(* Logix 5000 AddOnInstructionDefinition export Banner_QS18EAF_Param_v4; software revision 33.00; part 2 of 2 *)
(* tags used below, declared in another part *)
   QS18EAF : Banner_QS18EAF_v4;
   Port_Data : Banner_IOL_Port_v4;
   Port : DINT;
   Local_Control : DINT;
   Command_Being_Processed : BOOL;
   Update_Archive : BOOL;
   Index_Write_Inprocess : INT;
   Index_Write_Control : INT;
   Inprocess_Index : DINT;
(* Banner_QS18EAF_Param_v4, continued *)

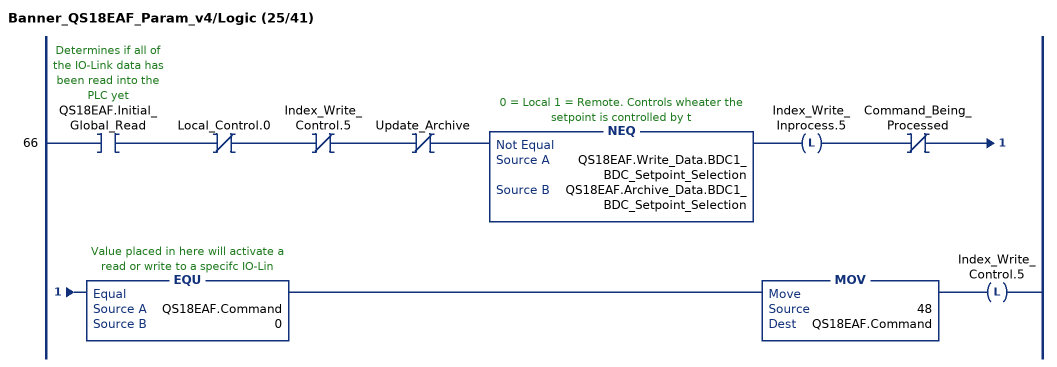
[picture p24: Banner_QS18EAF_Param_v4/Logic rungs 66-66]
   66: XIC(QS18EAF.Initial_Global_Read)XIO(Local_Control.0)XIO(Index_Write_Control.5)XIO(Update_Archive)NEQ(QS18EAF.Write_Data.BDC1_BDC_Setpoint_Selection,QS18EAF.Archive_Data.BDC1_BDC_Setpoint_Selection)OTL(Index_Write_Inprocess.5)XIO(Command_Being_Processed)EQU(QS18EAF.Command,0)MOV(48,QS18EAF.Command)OTL(Index_Write_Control.5);
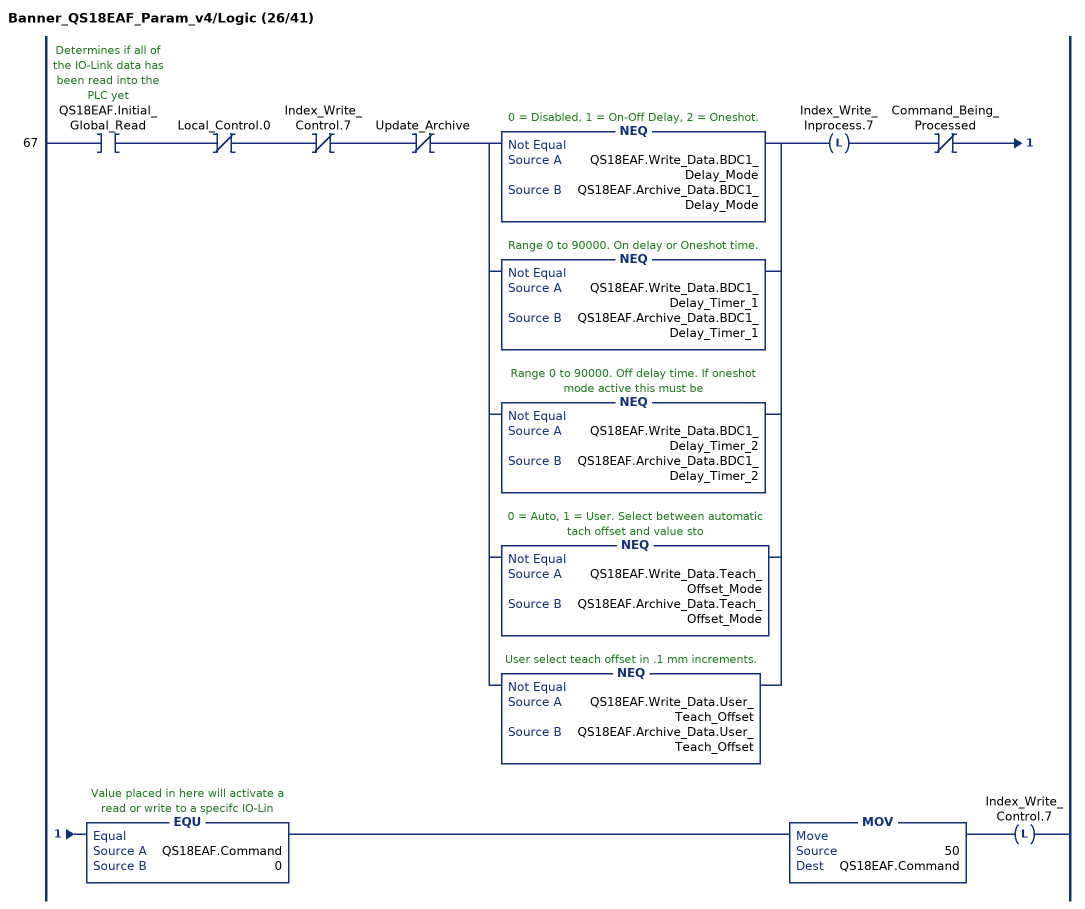
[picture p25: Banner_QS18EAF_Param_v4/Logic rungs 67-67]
   67: XIC(QS18EAF.Initial_Global_Read)XIO(Local_Control.0)XIO(Index_Write_Control.7)XIO(Update_Archive)[NEQ(QS18EAF.Write_Data.BDC1_Delay_Mode,QS18EAF.Archive_Data.BDC1_Delay_Mode) ,NEQ(QS18EAF.Write_Data.BDC1_Delay_Timer_1,QS18EAF.Archive_Data.BDC1_Delay_Timer_1) ,NEQ(QS18EAF.Write_Data.BDC1_Delay_Timer_2,QS18EAF.Archive_Data.BDC1_Delay_Timer_2) ,NEQ(QS18EAF.Write_Data.Teach_Offset_Mode,QS18EAF.Archive_Data.Teach_Offset_Mode) ,NEQ(QS18EAF.Write_Data.User_Teach_Offset,QS18EAF.Archive_Data.User_Teach_Offset) ]OTL(Index_Write_Inprocess.7)XIO(Command_Being_Processed)EQU(QS18EAF.Command,0)MOV(50,QS18EAF.Command)OTL(Index_Write_Control.7);
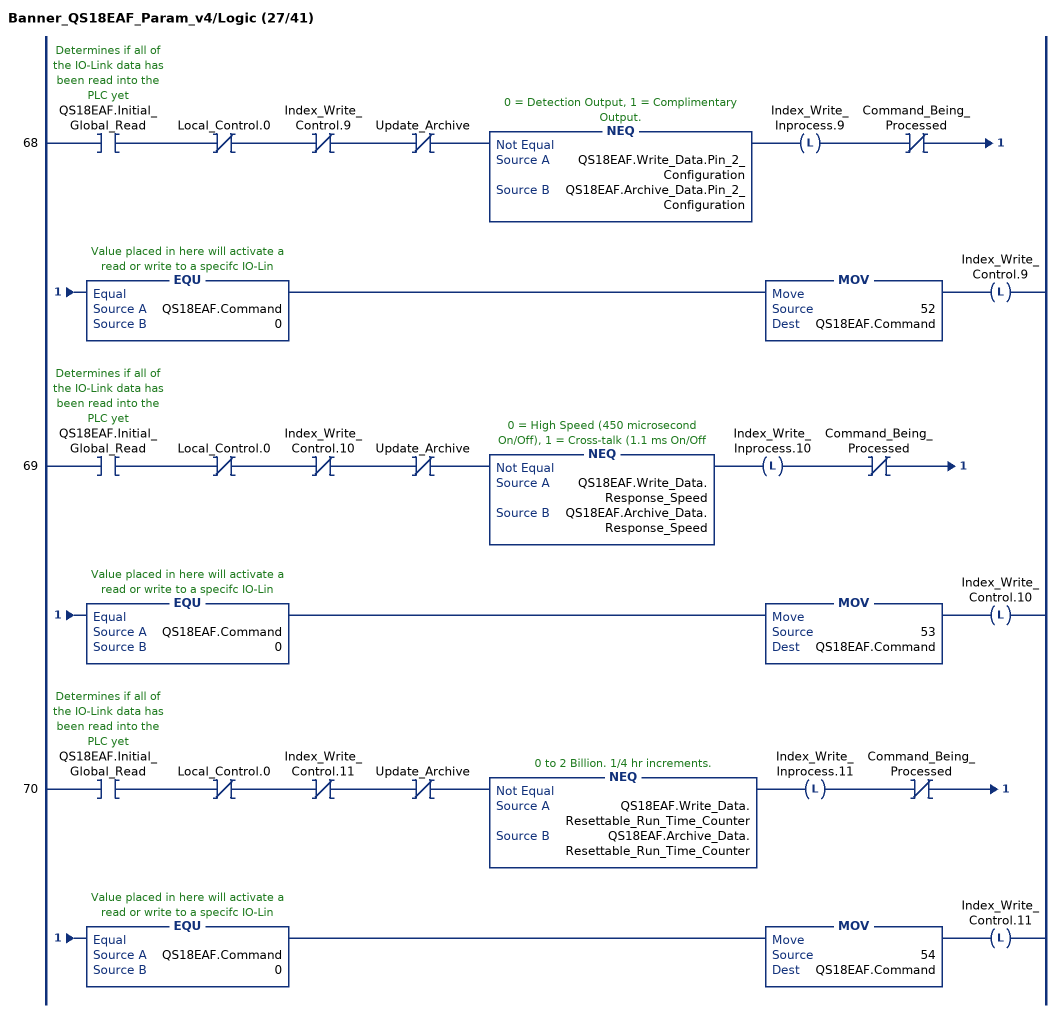
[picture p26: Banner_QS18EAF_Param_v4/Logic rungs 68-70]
   68: XIC(QS18EAF.Initial_Global_Read)XIO(Local_Control.0)XIO(Index_Write_Control.9)XIO(Update_Archive)NEQ(QS18EAF.Write_Data.Pin_2_Configuration,QS18EAF.Archive_Data.Pin_2_Configuration)OTL(Index_Write_Inprocess.9)XIO(Command_Being_Processed)EQU(QS18EAF.Command,0)MOV(52,QS18EAF.Command)OTL(Index_Write_Control.9);
   69: XIC(QS18EAF.Initial_Global_Read)XIO(Local_Control.0)XIO(Index_Write_Control.10)XIO(Update_Archive)NEQ(QS18EAF.Write_Data.Response_Speed,QS18EAF.Archive_Data.Response_Speed)OTL(Index_Write_Inprocess.10)XIO(Command_Being_Processed)EQU(QS18EAF.Command,0)MOV(53,QS18EAF.Command)OTL(Index_Write_Control.10);
   70: XIC(QS18EAF.Initial_Global_Read)XIO(Local_Control.0)XIO(Index_Write_Control.11)XIO(Update_Archive)NEQ(QS18EAF.Write_Data.Resettable_Run_Time_Counter,QS18EAF.Archive_Data.Resettable_Run_Time_Counter)OTL(Index_Write_Inprocess.11)XIO(Command_Being_Processed)EQU(QS18EAF.Command,0)MOV(54,QS18EAF.Command)OTL(Index_Write_Control.11);
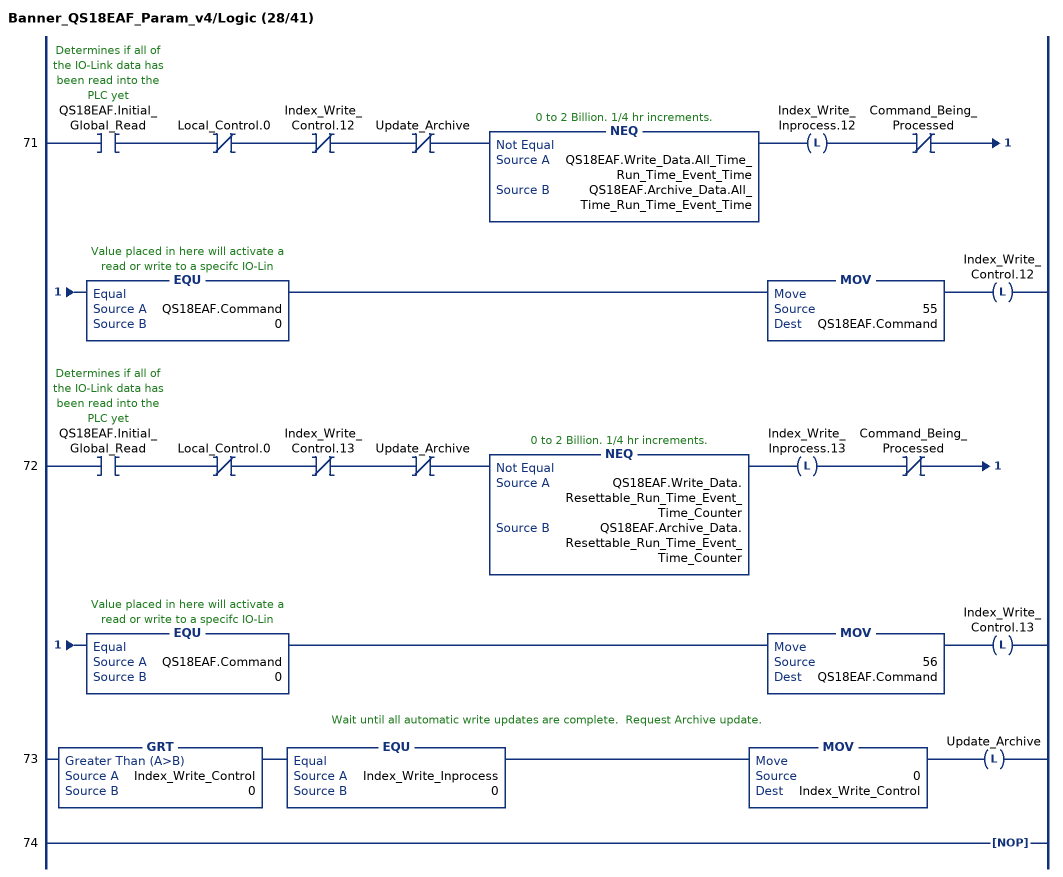
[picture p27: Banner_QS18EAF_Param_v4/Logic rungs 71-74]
   71: XIC(QS18EAF.Initial_Global_Read)XIO(Local_Control.0)XIO(Index_Write_Control.12)XIO(Update_Archive)NEQ(QS18EAF.Write_Data.All_Time_Run_Time_Event_Time,QS18EAF.Archive_Data.All_Time_Run_Time_Event_Time)OTL(Index_Write_Inprocess.12)XIO(Command_Being_Processed)EQU(QS18EAF.Command,0)MOV(55,QS18EAF.Command)OTL(Index_Write_Control.12);
   72: XIC(QS18EAF.Initial_Global_Read)XIO(Local_Control.0)XIO(Index_Write_Control.13)XIO(Update_Archive)NEQ(QS18EAF.Write_Data.Resettable_Run_Time_Event_Time_Counter,QS18EAF.Archive_Data.Resettable_Run_Time_Event_Time_Counter)OTL(Index_Write_Inprocess.13)XIO(Command_Being_Processed)EQU(QS18EAF.Command,0)MOV(56,QS18EAF.Command)OTL(Index_Write_Control.13);
   // Wait until all automatic write updates are complete.  Request Archive update.
   73: GRT(Index_Write_Control,0)EQU(Index_Write_Inprocess,0)MOV(0,Index_Write_Control)OTL(Update_Archive);
   74: NOP();
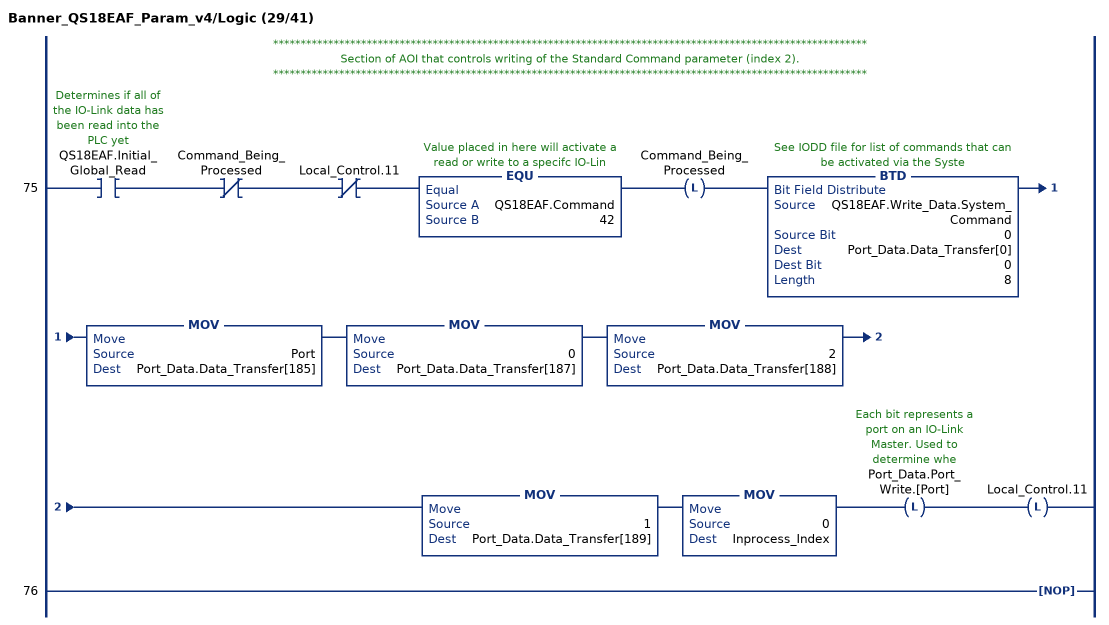
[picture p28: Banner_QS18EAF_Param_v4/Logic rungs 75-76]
   // ************************************************************************************************************
   // Section of AOI that controls writing of the Standard Command parameter (index 2).
   // ************************************************************************************************************
   75: XIC(QS18EAF.Initial_Global_Read)XIO(Command_Being_Processed)XIO(Local_Control.11)EQU(QS18EAF.Command,42)OTL(Command_Being_Processed)BTD(QS18EAF.Write_Data.System_Command,0,Port_Data.Data_Transfer[0],0,8)MOV(Port,Port_Data.Data_Transfer[185])MOV(0,Port_Data.Data_Transfer[187])MOV(2,Port_Data.Data_Transfer[188])MOV(1,Port_Data.Data_Transfer[189])MOV(0,Inprocess_Index)OTL(Port_Data.Port_Write.[Port])OTL(Local_Control.11);
   76: NOP();
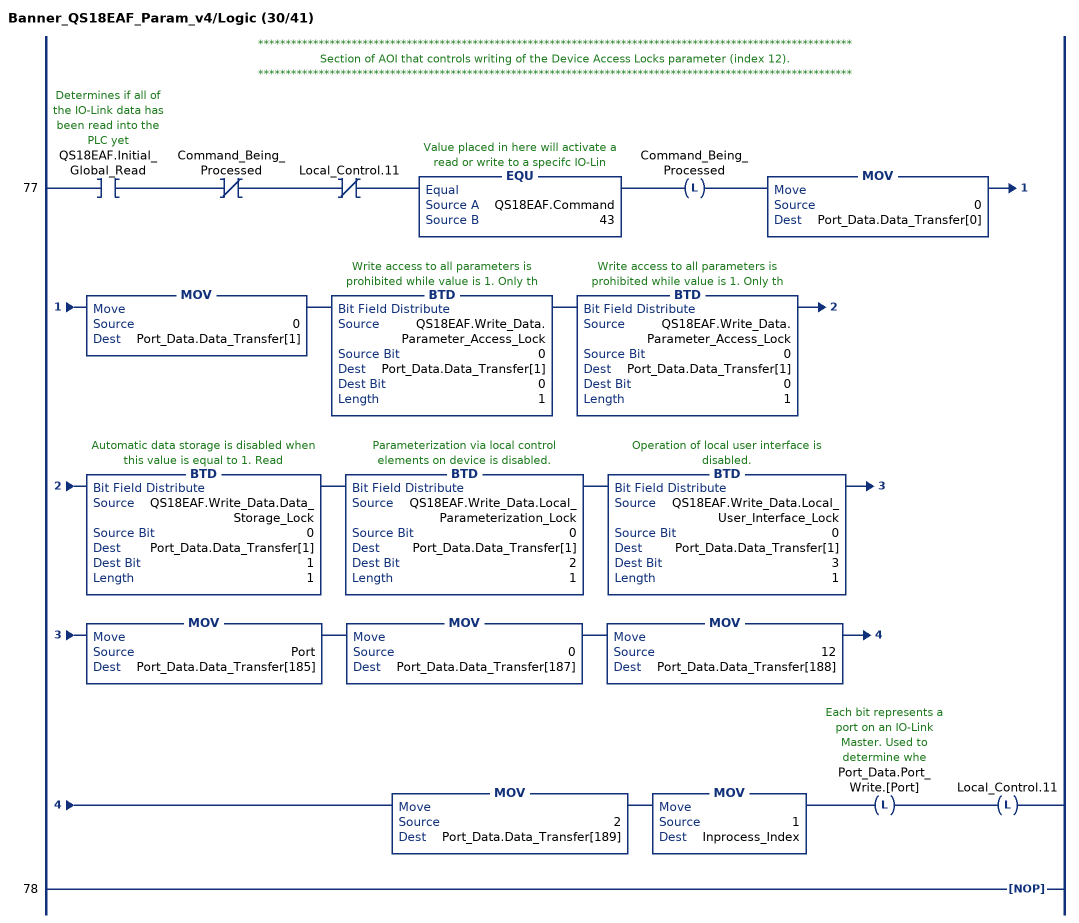
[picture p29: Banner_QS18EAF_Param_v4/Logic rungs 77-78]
   // ************************************************************************************************************
   // Section of AOI that controls writing of the Device Access Locks parameter (index 12).
   // ************************************************************************************************************
   77: XIC(QS18EAF.Initial_Global_Read)XIO(Command_Being_Processed)XIO(Local_Control.11)EQU(QS18EAF.Command,43)OTL(Command_Being_Processed)MOV(0,Port_Data.Data_Transfer[0])MOV(0,Port_Data.Data_Transfer[1])BTD(QS18EAF.Write_Data.Parameter_Access_Lock,0,Port_Data.Data_Transfer[1],0,1)BTD(QS18EAF.Write_Data.Parameter_Access_Lock,0,Port_Data.Data_Transfer[1],0,1)BTD(QS18EAF.Write_Data.Data_Storage_Lock,0,Port_Data.Data_Transfer[1],1,1)BTD(QS18EAF.Write_Data.Local_Parameterization_Lock,0,Port_Data.Data_Transfer[1],2,1)BTD(QS18EAF.Write_Data.Local_User_Interface_Lock,0,Port_Data.Data_Transfer[1],3,1)MOV(Port,Port_Data.Data_Transfer[185])MOV(0,Port_Data.Data_Transfer[187])MOV(12,Port_Data.Data_Transfer[188])MOV(2,Port_Data.Data_Transfer[189])MOV(1,Inprocess_Index)OTL(Port_Data.Port_Write.[Port])OTL(Local_Control.11);
   78: NOP();
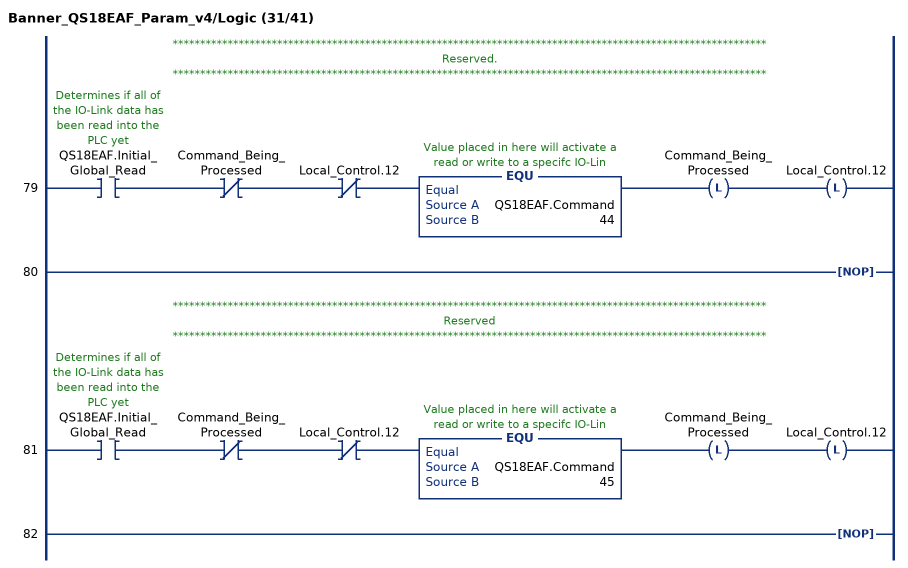
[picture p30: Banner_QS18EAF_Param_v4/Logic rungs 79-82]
   // ************************************************************************************************************
   // Reserved.
   // ************************************************************************************************************
   79: XIC(QS18EAF.Initial_Global_Read)XIO(Command_Being_Processed)XIO(Local_Control.12)EQU(QS18EAF.Command,44)OTL(Command_Being_Processed)OTL(Local_Control.12);
   80: NOP();
   // ************************************************************************************************************
   // Reserved
   // ************************************************************************************************************
   81: XIC(QS18EAF.Initial_Global_Read)XIO(Command_Being_Processed)XIO(Local_Control.12)EQU(QS18EAF.Command,45)OTL(Command_Being_Processed)OTL(Local_Control.12);
   82: NOP();
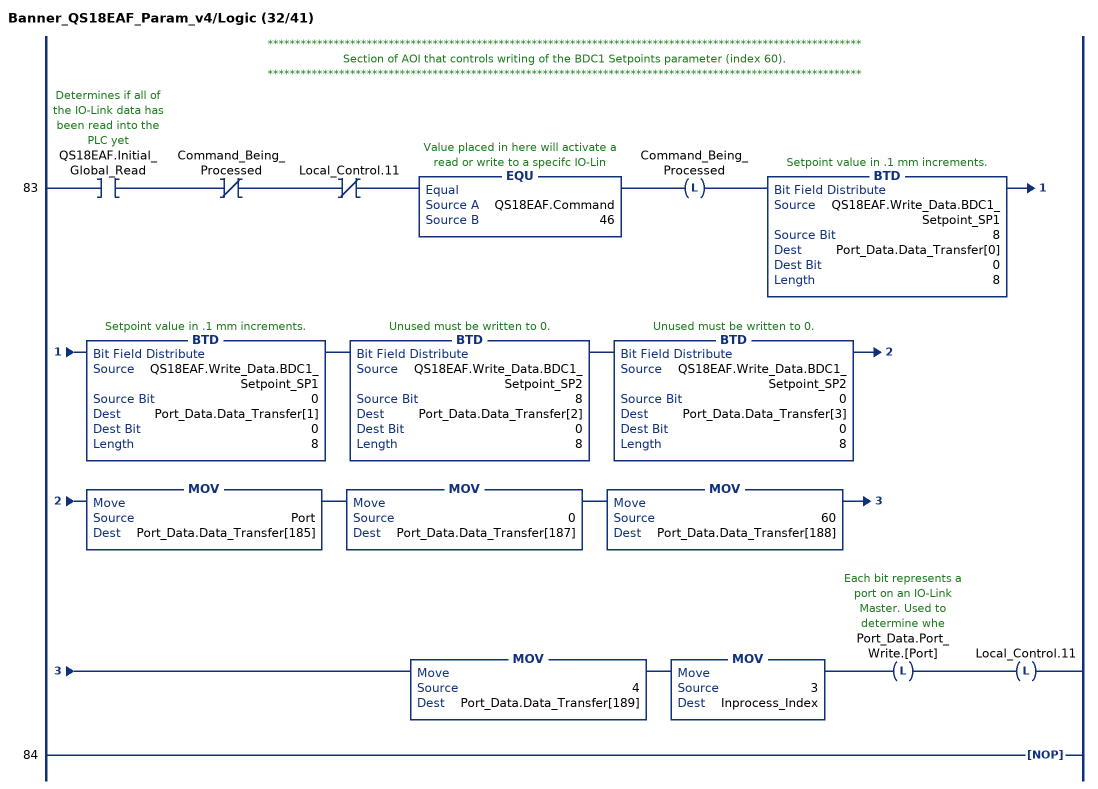
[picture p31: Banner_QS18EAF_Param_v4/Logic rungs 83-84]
   // ************************************************************************************************************
   // Section of AOI that controls writing of the BDC1 Setpoints parameter (index 60).
   // ************************************************************************************************************
   83: XIC(QS18EAF.Initial_Global_Read)XIO(Command_Being_Processed)XIO(Local_Control.11)EQU(QS18EAF.Command,46)OTL(Command_Being_Processed)BTD(QS18EAF.Write_Data.BDC1_Setpoint_SP1,8,Port_Data.Data_Transfer[0],0,8)BTD(QS18EAF.Write_Data.BDC1_Setpoint_SP1,0,Port_Data.Data_Transfer[1],0,8)BTD(QS18EAF.Write_Data.BDC1_Setpoint_SP2,8,Port_Data.Data_Transfer[2],0,8)BTD(QS18EAF.Write_Data.BDC1_Setpoint_SP2,0,Port_Data.Data_Transfer[3],0,8)MOV(Port,Port_Data.Data_Transfer[185])MOV(0,Port_Data.Data_Transfer[187])MOV(60,Port_Data.Data_Transfer[188])MOV(4,Port_Data.Data_Transfer[189])MOV(3,Inprocess_Index)OTL(Port_Data.Port_Write.[Port])OTL(Local_Control.11);
   84: NOP();
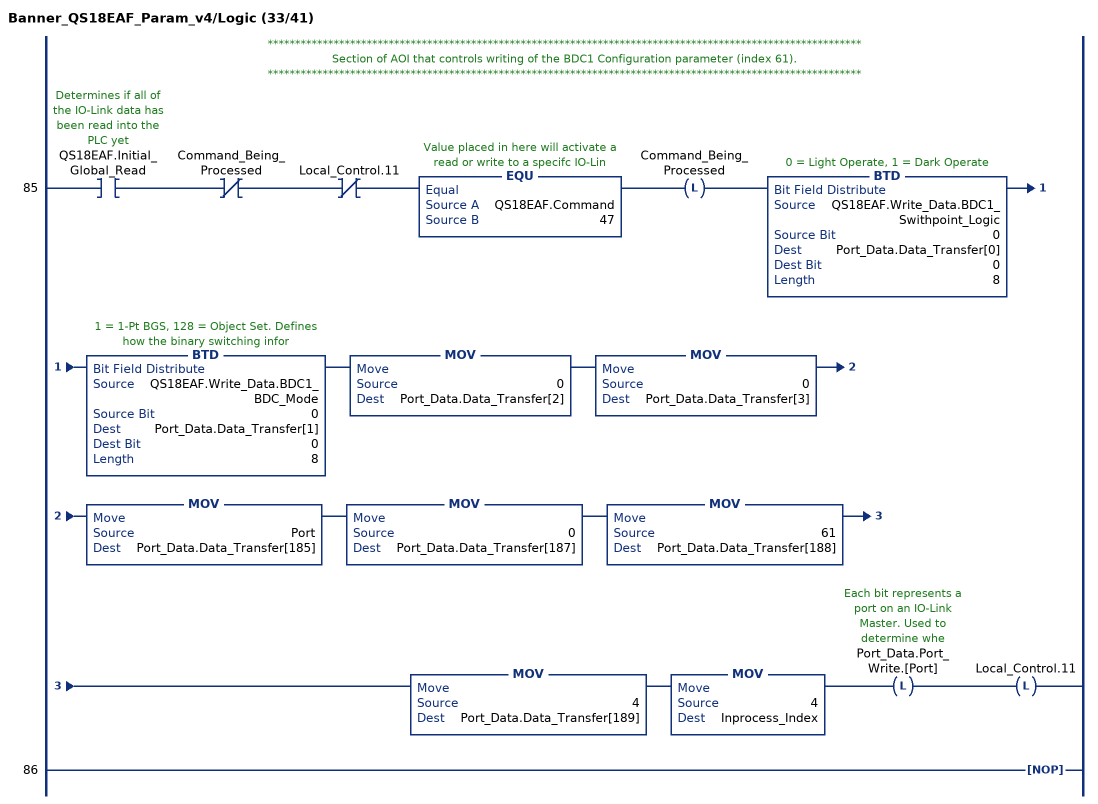
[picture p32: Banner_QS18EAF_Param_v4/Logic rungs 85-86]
   // ************************************************************************************************************
   // Section of AOI that controls writing of the BDC1 Configuration parameter (index 61).
   // ************************************************************************************************************
   85: XIC(QS18EAF.Initial_Global_Read)XIO(Command_Being_Processed)XIO(Local_Control.11)EQU(QS18EAF.Command,47)OTL(Command_Being_Processed)BTD(QS18EAF.Write_Data.BDC1_Swithpoint_Logic,0,Port_Data.Data_Transfer[0],0,8)BTD(QS18EAF.Write_Data.BDC1_BDC_Mode,0,Port_Data.Data_Transfer[1],0,8)MOV(0,Port_Data.Data_Transfer[2])MOV(0,Port_Data.Data_Transfer[3])MOV(Port,Port_Data.Data_Transfer[185])MOV(0,Port_Data.Data_Transfer[187])MOV(61,Port_Data.Data_Transfer[188])MOV(4,Port_Data.Data_Transfer[189])MOV(4,Inprocess_Index)OTL(Port_Data.Port_Write.[Port])OTL(Local_Control.11);
   86: NOP();
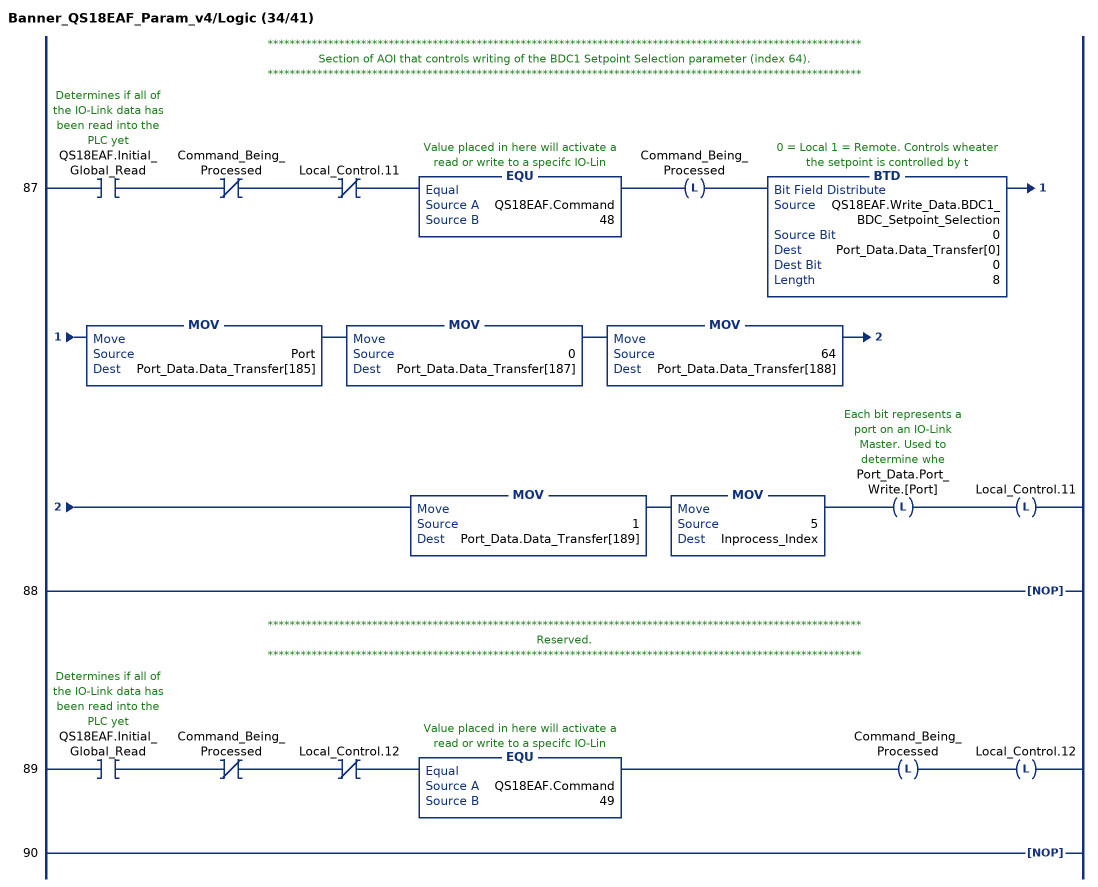
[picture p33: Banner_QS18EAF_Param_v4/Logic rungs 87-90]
   // ************************************************************************************************************
   // Section of AOI that controls writing of the BDC1 Setpoint Selection parameter (index 64).
   // ************************************************************************************************************
   87: XIC(QS18EAF.Initial_Global_Read)XIO(Command_Being_Processed)XIO(Local_Control.11)EQU(QS18EAF.Command,48)OTL(Command_Being_Processed)BTD(QS18EAF.Write_Data.BDC1_BDC_Setpoint_Selection,0,Port_Data.Data_Transfer[0],0,8)MOV(Port,Port_Data.Data_Transfer[185])MOV(0,Port_Data.Data_Transfer[187])MOV(64,Port_Data.Data_Transfer[188])MOV(1,Port_Data.Data_Transfer[189])MOV(5,Inprocess_Index)OTL(Port_Data.Port_Write.[Port])OTL(Local_Control.11);
   88: NOP();
   // ************************************************************************************************************
   // Reserved.
   // ************************************************************************************************************
   89: XIC(QS18EAF.Initial_Global_Read)XIO(Command_Being_Processed)XIO(Local_Control.12)EQU(QS18EAF.Command,49)OTL(Command_Being_Processed)OTL(Local_Control.12);
   90: NOP();
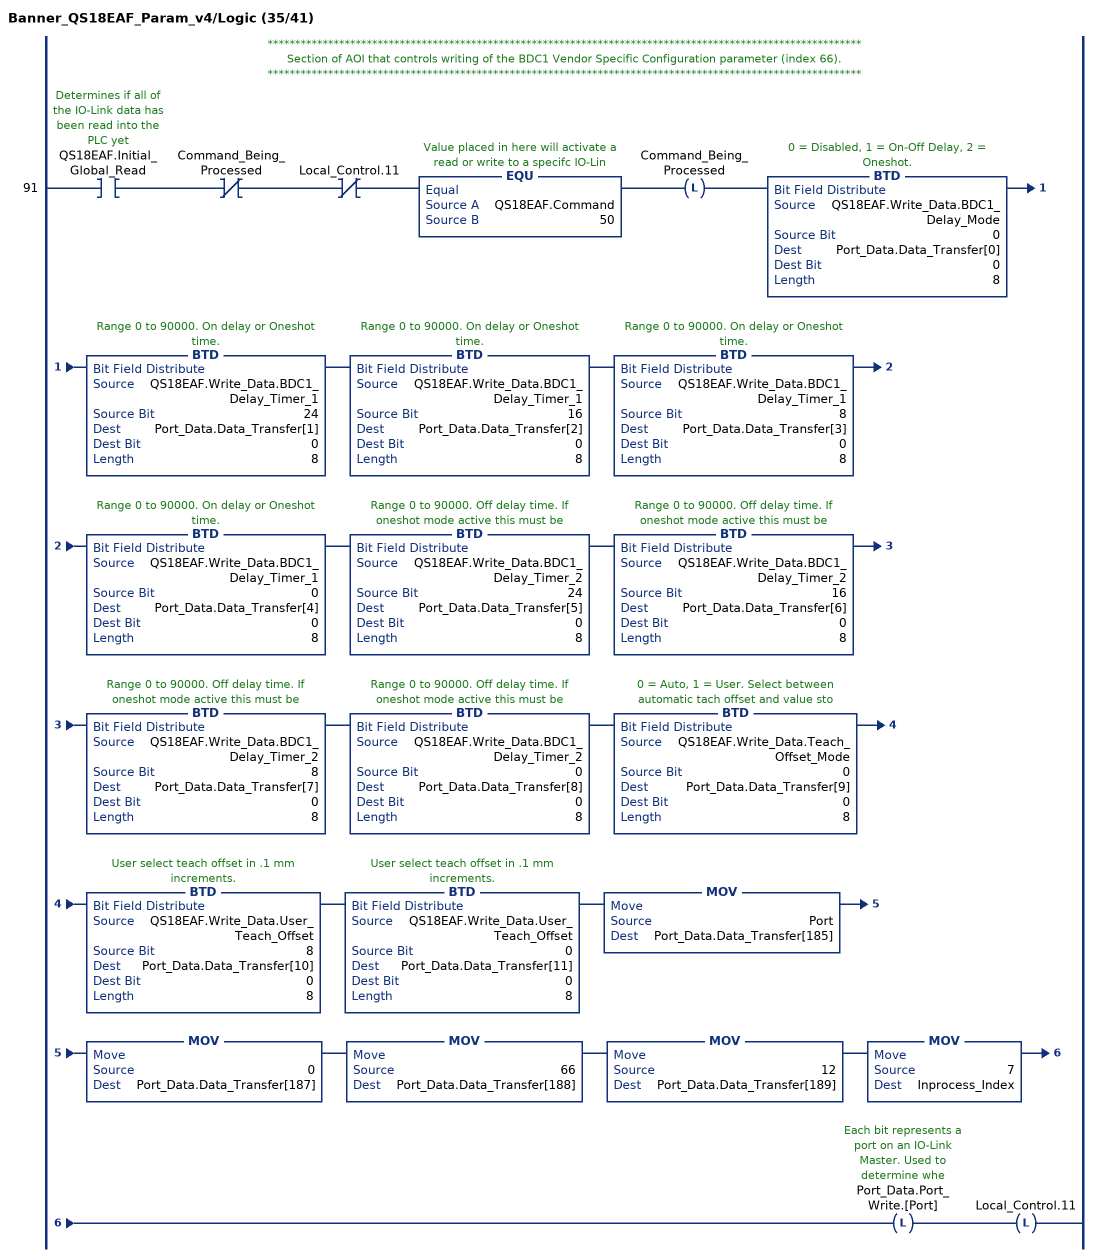
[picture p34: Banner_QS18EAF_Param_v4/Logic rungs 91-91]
   // ************************************************************************************************************
   // Section of AOI that controls writing of the BDC1 Vendor Specific Configuration parameter (index 66).
   // ************************************************************************************************************
   91: XIC(QS18EAF.Initial_Global_Read)XIO(Command_Being_Processed)XIO(Local_Control.11)EQU(QS18EAF.Command,50)OTL(Command_Being_Processed)BTD(QS18EAF.Write_Data.BDC1_Delay_Mode,0,Port_Data.Data_Transfer[0],0,8)BTD(QS18EAF.Write_Data.BDC1_Delay_Timer_1,24,Port_Data.Data_Transfer[1],0,8)BTD(QS18EAF.Write_Data.BDC1_Delay_Timer_1,16,Port_Data.Data_Transfer[2],0,8)BTD(QS18EAF.Write_Data.BDC1_Delay_Timer_1,8,Port_Data.Data_Transfer[3],0,8)BTD(QS18EAF.Write_Data.BDC1_Delay_Timer_1,0,Port_Data.Data_Transfer[4],0,8)BTD(QS18EAF.Write_Data.BDC1_Delay_Timer_2,24,Port_Data.Data_Transfer[5],0,8)BTD(QS18EAF.Write_Data.BDC1_Delay_Timer_2,16,Port_Data.Data_Transfer[6],0,8)BTD(QS18EAF.Write_Data.BDC1_Delay_Timer_2,8,Port_Data.Data_Transfer[7],0,8)BTD(QS18EAF.Write_Data.BDC1_Delay_Timer_2,0,Port_Data.Data_Transfer[8],0,8)BTD(QS18EAF.Write_Data.Teach_Offset_Mode,0,Port_Data.Data_Transfer[9],0,8)BTD(QS18EAF.Write_Data.User_Teach_Offset,8,Port_Data.Data_Transfer[10],0,8)BTD(QS18EAF.Write_Data.User_Teach_Offset,0,Port_Data.Data_Transfer[11],0,8)MOV(Port,Port_Data.Data_Transfer[185])MOV(0,Port_Data.Data_Transfer[187])MOV(66,Port_Data.Data_Transfer[188])MOV(12,Port_Data.Data_Transfer[189])MOV(7,Inprocess_Index)OTL(Port_Data.Port_Write.[Port])OTL(Local_Control.11);
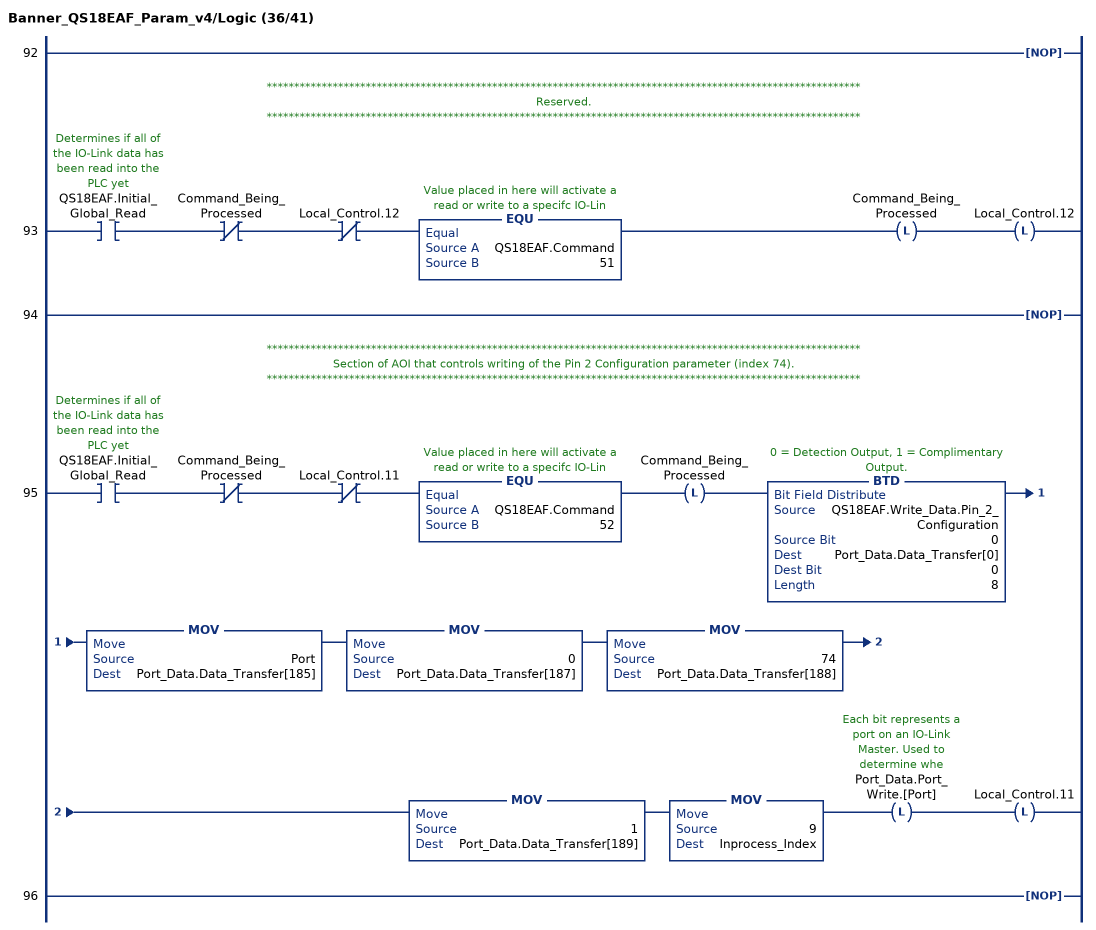
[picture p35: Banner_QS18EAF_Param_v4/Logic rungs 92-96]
   92: NOP();
   // ************************************************************************************************************
   // Reserved.
   // ************************************************************************************************************
   93: XIC(QS18EAF.Initial_Global_Read)XIO(Command_Being_Processed)XIO(Local_Control.12)EQU(QS18EAF.Command,51)OTL(Command_Being_Processed)OTL(Local_Control.12);
   94: NOP();
   // ************************************************************************************************************
   // Section of AOI that controls writing of the Pin 2 Configuration parameter (index 74).
   // ************************************************************************************************************
   95: XIC(QS18EAF.Initial_Global_Read)XIO(Command_Being_Processed)XIO(Local_Control.11)EQU(QS18EAF.Command,52)OTL(Command_Being_Processed)BTD(QS18EAF.Write_Data.Pin_2_Configuration,0,Port_Data.Data_Transfer[0],0,8)MOV(Port,Port_Data.Data_Transfer[185])MOV(0,Port_Data.Data_Transfer[187])MOV(74,Port_Data.Data_Transfer[188])MOV(1,Port_Data.Data_Transfer[189])MOV(9,Inprocess_Index)OTL(Port_Data.Port_Write.[Port])OTL(Local_Control.11);
   96: NOP();
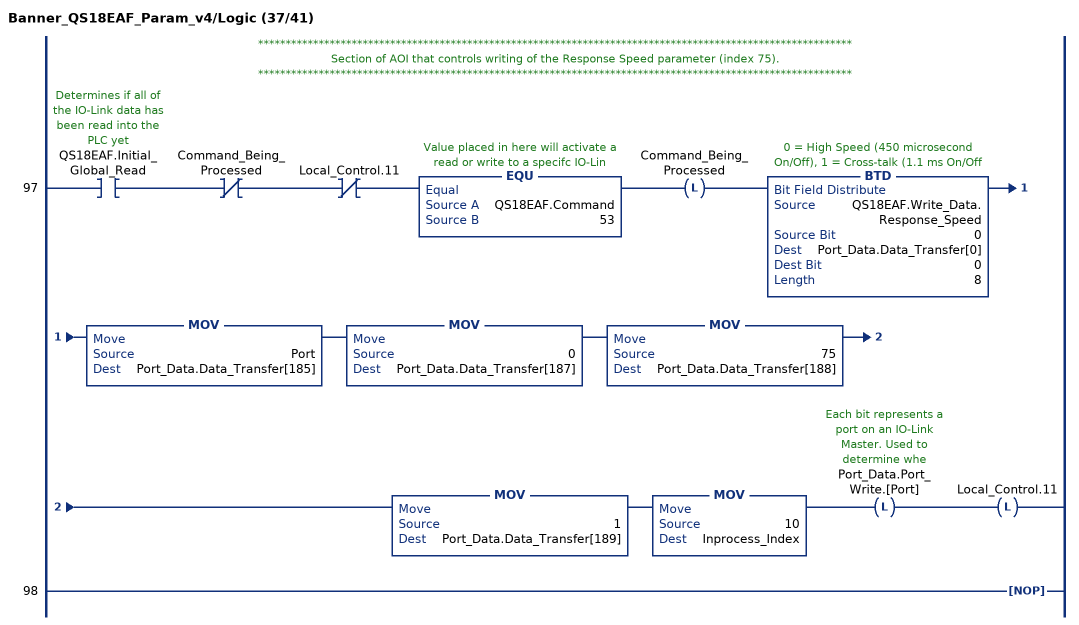
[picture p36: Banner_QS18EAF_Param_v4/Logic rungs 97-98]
   // ************************************************************************************************************
   // Section of AOI that controls writing of the Response Speed parameter (index 75).
   // ************************************************************************************************************
   97: XIC(QS18EAF.Initial_Global_Read)XIO(Command_Being_Processed)XIO(Local_Control.11)EQU(QS18EAF.Command,53)OTL(Command_Being_Processed)BTD(QS18EAF.Write_Data.Response_Speed,0,Port_Data.Data_Transfer[0],0,8)MOV(Port,Port_Data.Data_Transfer[185])MOV(0,Port_Data.Data_Transfer[187])MOV(75,Port_Data.Data_Transfer[188])MOV(1,Port_Data.Data_Transfer[189])MOV(10,Inprocess_Index)OTL(Port_Data.Port_Write.[Port])OTL(Local_Control.11);
   98: NOP();
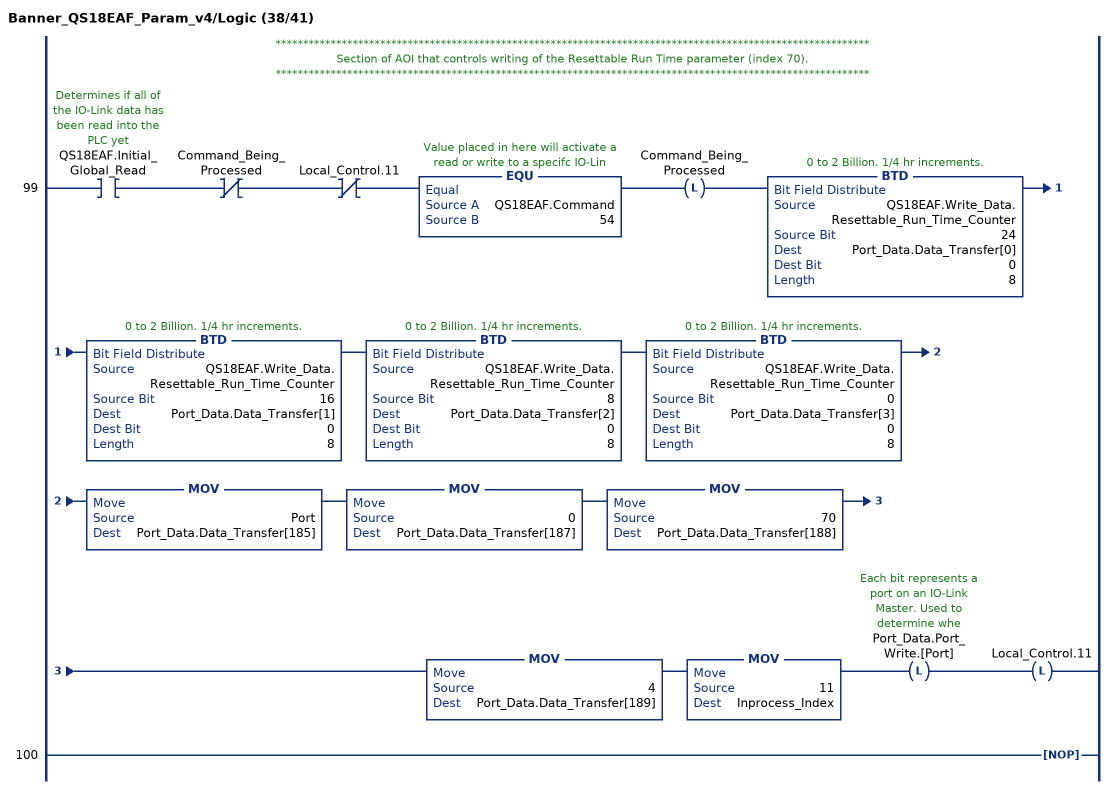
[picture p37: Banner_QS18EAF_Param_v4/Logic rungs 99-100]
   // ************************************************************************************************************
   // Section of AOI that controls writing of the Resettable Run Time parameter (index 70).
   // ************************************************************************************************************
   99: XIC(QS18EAF.Initial_Global_Read)XIO(Command_Being_Processed)XIO(Local_Control.11)EQU(QS18EAF.Command,54)OTL(Command_Being_Processed)BTD(QS18EAF.Write_Data.Resettable_Run_Time_Counter,24,Port_Data.Data_Transfer[0],0,8)BTD(QS18EAF.Write_Data.Resettable_Run_Time_Counter,16,Port_Data.Data_Transfer[1],0,8)BTD(QS18EAF.Write_Data.Resettable_Run_Time_Counter,8,Port_Data.Data_Transfer[2],0,8)BTD(QS18EAF.Write_Data.Resettable_Run_Time_Counter,0,Port_Data.Data_Transfer[3],0,8)MOV(Port,Port_Data.Data_Transfer[185])MOV(0,Port_Data.Data_Transfer[187])MOV(70,Port_Data.Data_Transfer[188])MOV(4,Port_Data.Data_Transfer[189])MOV(11,Inprocess_Index)OTL(Port_Data.Port_Write.[Port])OTL(Local_Control.11);
   100: NOP();
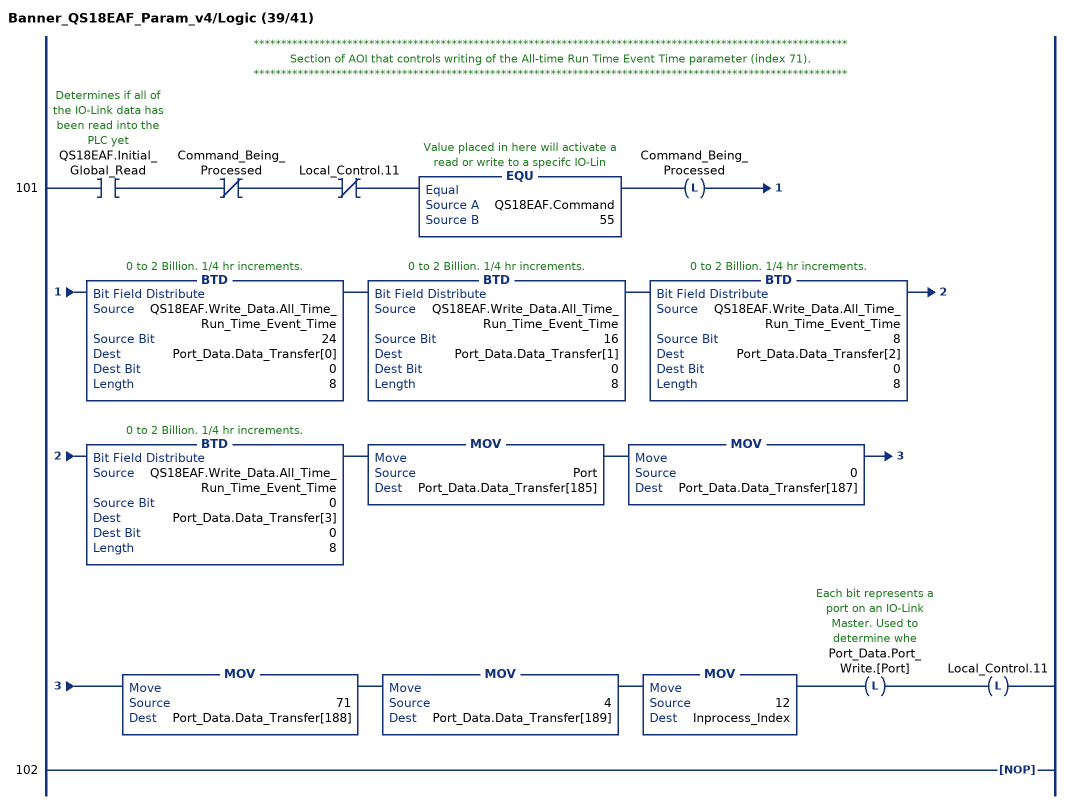
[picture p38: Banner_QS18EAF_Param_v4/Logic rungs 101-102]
   // ************************************************************************************************************
   // Section of AOI that controls writing of the All-time Run Time Event Time parameter (index 71).
   // ************************************************************************************************************
   101: XIC(QS18EAF.Initial_Global_Read)XIO(Command_Being_Processed)XIO(Local_Control.11)EQU(QS18EAF.Command,55)OTL(Command_Being_Processed)BTD(QS18EAF.Write_Data.All_Time_Run_Time_Event_Time,24,Port_Data.Data_Transfer[0],0,8)BTD(QS18EAF.Write_Data.All_Time_Run_Time_Event_Time,16,Port_Data.Data_Transfer[1],0,8)BTD(QS18EAF.Write_Data.All_Time_Run_Time_Event_Time,8,Port_Data.Data_Transfer[2],0,8)BTD(QS18EAF.Write_Data.All_Time_Run_Time_Event_Time,0,Port_Data.Data_Transfer[3],0,8)MOV(Port,Port_Data.Data_Transfer[185])MOV(0,Port_Data.Data_Transfer[187])MOV(71,Port_Data.Data_Transfer[188])MOV(4,Port_Data.Data_Transfer[189])MOV(12,Inprocess_Index)OTL(Port_Data.Port_Write.[Port])OTL(Local_Control.11);
   102: NOP();
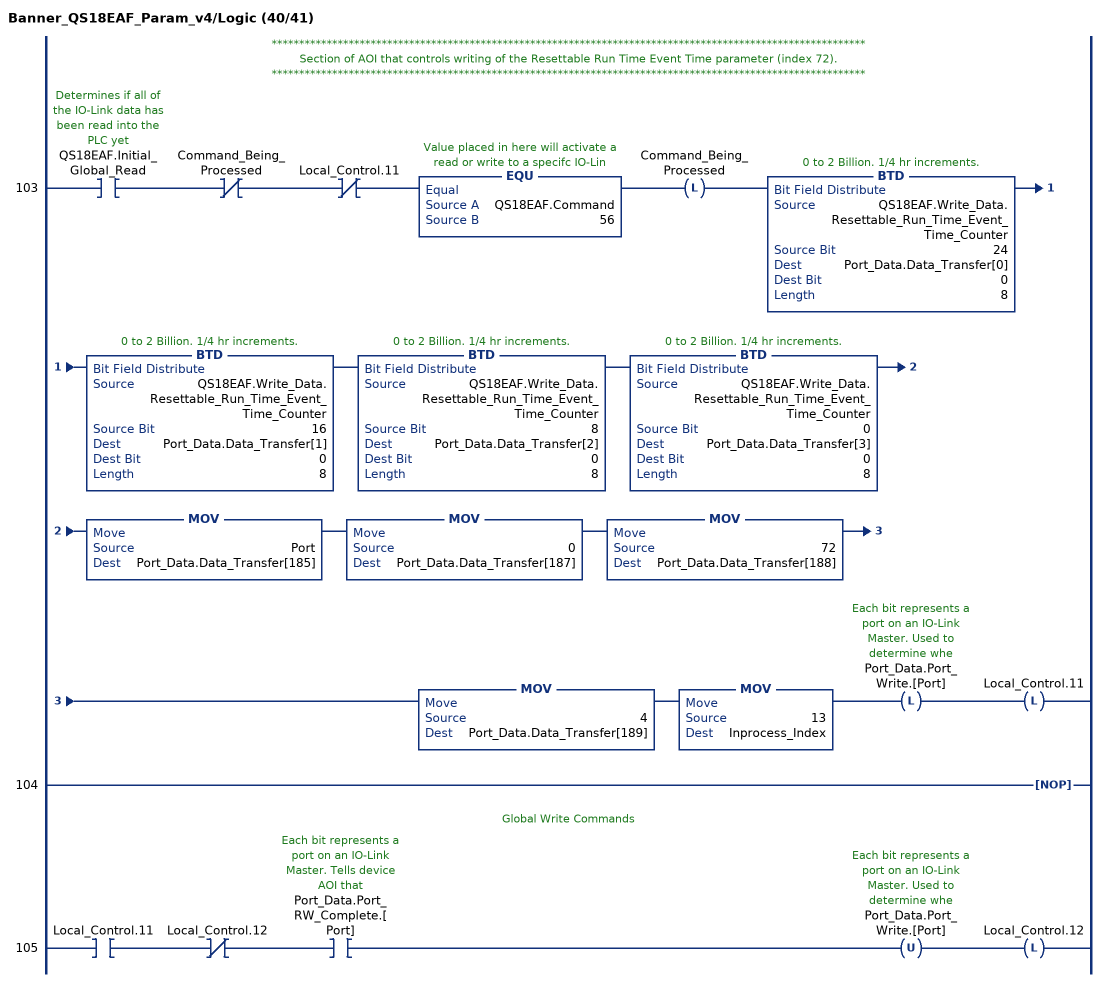
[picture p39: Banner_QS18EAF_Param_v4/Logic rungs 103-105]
   // ************************************************************************************************************
   // Section of AOI that controls writing of the Resettable Run Time Event Time parameter (index 72).
   // ************************************************************************************************************
   103: XIC(QS18EAF.Initial_Global_Read)XIO(Command_Being_Processed)XIO(Local_Control.11)EQU(QS18EAF.Command,56)OTL(Command_Being_Processed)BTD(QS18EAF.Write_Data.Resettable_Run_Time_Event_Time_Counter,24,Port_Data.Data_Transfer[0],0,8)BTD(QS18EAF.Write_Data.Resettable_Run_Time_Event_Time_Counter,16,Port_Data.Data_Transfer[1],0,8)BTD(QS18EAF.Write_Data.Resettable_Run_Time_Event_Time_Counter,8,Port_Data.Data_Transfer[2],0,8)BTD(QS18EAF.Write_Data.Resettable_Run_Time_Event_Time_Counter,0,Port_Data.Data_Transfer[3],0,8)MOV(Port,Port_Data.Data_Transfer[185])MOV(0,Port_Data.Data_Transfer[187])MOV(72,Port_Data.Data_Transfer[188])MOV(4,Port_Data.Data_Transfer[189])MOV(13,Inprocess_Index)OTL(Port_Data.Port_Write.[Port])OTL(Local_Control.11);
   104: NOP();
   // Global Write Commands
   105: XIC(Local_Control.11)XIO(Local_Control.12)XIC(Port_Data.Port_RW_Complete.[Port])OTU(Port_Data.Port_Write.[Port])OTL(Local_Control.12);
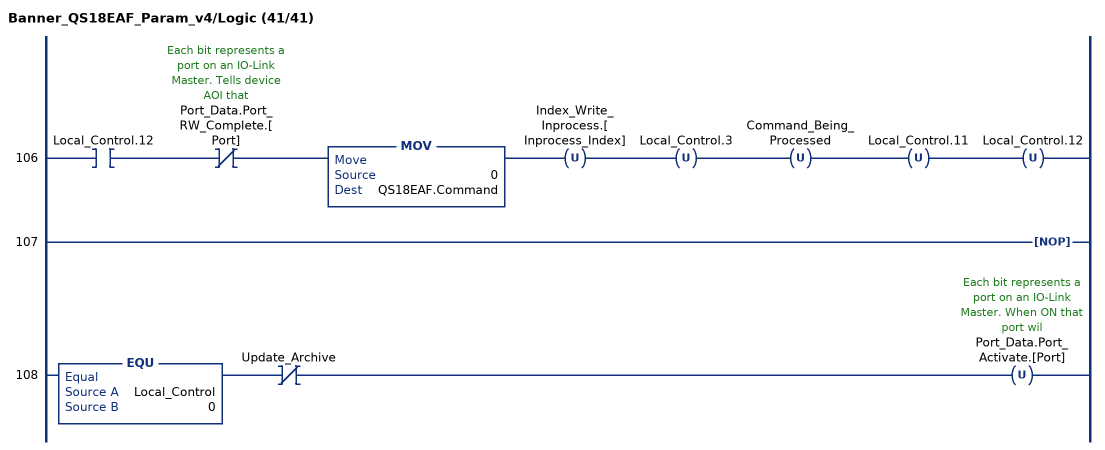
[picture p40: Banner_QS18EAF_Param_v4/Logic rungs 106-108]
   106: XIC(Local_Control.12)XIO(Port_Data.Port_RW_Complete.[Port])MOV(0,QS18EAF.Command)OTU(Index_Write_Inprocess.[Inprocess_Index])OTU(Local_Control.3)OTU(Command_Being_Processed)OTU(Local_Control.11)OTU(Local_Control.12);
   107: NOP();
   108: EQU(Local_Control,0)XIO(Update_Archive)OTU(Port_Data.Port_Activate.[Port]);
END_ROUTINE
END_ADD_ON_INSTRUCTION
